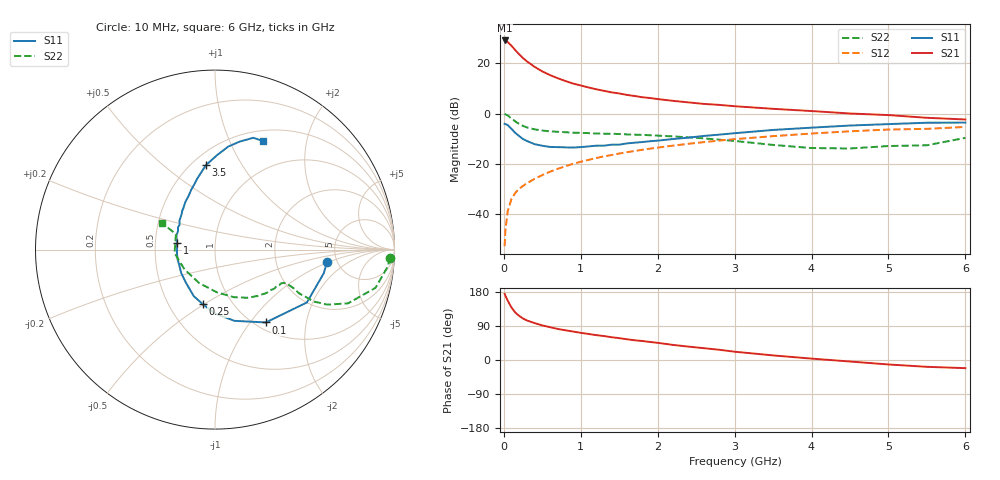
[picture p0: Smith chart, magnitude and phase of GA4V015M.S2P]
! Infineon Technologies  Discrete & RF Semiconductors
! BF775
! Si NPN RF Bipolar Junction Transistor in SOT23
! VCE = 4 V  IC = 15 mA
! Common Emitter S-Parameters:  May  1996
# GHz  S  MA  R  50
!  f  S11  S21  S12  S22
! GHz  MAG  ANG  MAG  ANG  MAG  ANG  MAG  ANG
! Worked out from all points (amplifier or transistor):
!   36 points, 10 MHz to 6 GHz, reference 50 ohm
!   highest |S21| = 29.1 dB at 10 MHz (marker M1)
!   |S21| within 3 dB of that: start of sweep to 124.5 MHz
!   unconditionally stable (mu >= 1): 469.3 MHz to 3.013 GHz
!   at 250 MHz: K = 0.79, MSG = 25.4 dB, |S12| = -28.8 dB
!   at 1.4 GHz: K = 1.10, MAG = 10.5 dB, |S12| = -16.5 dB
!   at 6 GHz: K = 0.95, MSG = 1.5 dB, |S12| = -5.3 dB
!   S11 on the Smith chart (normalised r, x): 10 MHz: 4.14, -0.96; 100 MHz: 1.11, -1.20; 250 MHz: 0.73, -0.49; 1 GHz: 0.65, +0.05; 3.5 GHz: 0.59, +0.71; 6 GHz: 0.63, +1.35
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0.01  0.6278 -6.4  28.55 174.8  0.0023 88.5  0.9778 -2.6
0.02  0.62 -12.3  28.15 169.9  0.0047 83.6  0.9664 -5.7
0.05  0.5907 -29.9  26.58 156.6  0.0114 76.6  0.9195 -13.4
0.1  0.4949 -55.1  22.36 138.4  0.0202 69.3  0.7993 -22.0
0.15  0.4115 -74.7  18.19 125.0  0.0266 65.4  0.6966 -26.1
0.2  0.3565 -90.0  15.13 116.3  0.0319 64.6  0.6226 -27.7
0.25  0.3107 -102.9  12.69 109.4  0.0365 64.6  0.5679 -27.5
0.3  0.2852 -114.4  10.95 104.3  0.0411 65.9  0.53 -27.5
0.4  0.2464 -130.8  8.521 97.4  0.0503 67.0  0.4855 -26.1
0.5  0.2291 -145.2  6.911 91.3  0.0598 67.7  0.4608 -25.7
0.6  0.217 -156.7  5.836 86.6  0.0697 68.0  0.4431 -25.4
0.7  0.2153 -165.9  5.065 82.0  0.0796 68.4  0.4347 -25.6
0.9  0.211 178.7  3.963 75.1  0.1002 67.8  0.4171 -26.7
1  0.2155 169.7  3.626 71.7  0.1101 67.3  0.4132 -27.2
1.1  0.2222 164.1  3.314 68.7  0.1198 66.9  0.409 -28.9
1.4  0.2408 148.8  2.647 60.1  0.1499 64.6  0.3968 -32.8
1.6  0.2553 140.7  2.354 54.7  0.1705 62.8  0.3857 -35.5
2.2  0.3121 122.1  1.794 39.8  0.2307 56.6  0.352 -47.0
3.5  0.4727 96.2  1.245 12.1  0.3559 40.8  0.2382 -87.4
4.5  0.5786 82.7  1.005 -4.0  0.4446 27.7  0.2023 -146.8
5.5  0.6584 71.1  0.825 -18.0  0.4972 12.8  0.2342 158.4
6  0.6614 65.9  0.764 -21.5  0.5428 8.7  0.3292 153.4
